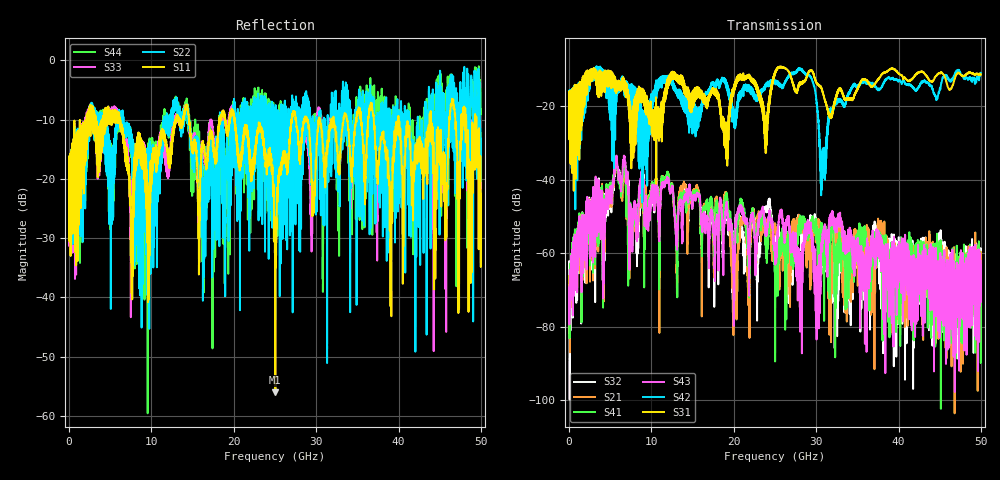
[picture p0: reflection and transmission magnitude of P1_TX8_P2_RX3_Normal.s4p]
!Keysight Technologies,N5225B,MY57041031,A.13.20.10
!Date: Friday, May 31, 2019 11:32:16
!Correction: S11(Full 4 Port(1,2,3,4))
!S12(Full 4 Port(1,2,3,4))
!S13(Full 4 Port(1,2,3,4))
!S14(Full 4 Port(1,2,3,4))
!S21(Full 4 Port(1,2,3,4))
!S22(Full 4 Port(1,2,3,4))
!S23(Full 4 Port(1,2,3,4))
!S24(Full 4 Port(1,2,3,4))
!S31(Full 4 Port(1,2,3,4))
!S32(Full 4 Port(1,2,3,4))
!S33(Full 4 Port(1,2,3,4))
!S34(Full 4 Port(1,2,3,4))
!S41(Full 4 Port(1,2,3,4))
!S42(Full 4 Port(1,2,3,4))
!S43(Full 4 Port(1,2,3,4))
!S44(Full 4 Port(1,2,3,4))
!S4P File: Measurements: <S11,S12,S13,S14>,
!<S21,S22,S23,S24>,
!<S31,S32,S33,S34>,
!<S41,S42,S43,S44>:
# Hz S  dB  R 50.0
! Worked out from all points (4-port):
!   5000 points, 10 MHz to 50 GHz, reference 50 ohm
!   strongest paths, dB at 10 MHz, 12.51 GHz, 25.01 GHz, 37.51 GHz, 50 GHz:
!     S31: -19.6, -10.8, -11.0, -12.6, -11.3
!     S42: -19.3, -14.2, -13.1, -15.6, -10.9
!     S43: -76.3, -42.0, -61.9, -55.2, -67.4
!     S41: -70.7, -41.7, -68.8, -59.2, -73.5
!     S21: -66.2, -42.0, -51.9, -52.8, -64.3
!     S32: -68.9, -41.5, -57.0, -62.4, -66.8
!   lowest |S11| = -56.0 dB at 25.05 GHz (marker M1), VSWR 1.00, Z = 49.8 - j0.000148 ohm
!   |S11| at or under -10 dB: 6.192 GHz to 12.89 GHz (6.696 GHz wide, 70.2 % of centre); 20.1 GHz to 26.99 GHz (6.893 GHz wide, 29.3 % of centre); 40 GHz to 43.77 GHz (3.764 GHz wide, 8.99 % of centre)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
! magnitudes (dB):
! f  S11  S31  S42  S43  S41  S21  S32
! 10 MHz  -19.5  -19.6  -19.3  -76.3  -70.7  -66.2  -68.9
! 5.71 GHz  -9.5  -15.2  -16.9  -34.8  -35.0  -35.4  -35.6
! 19.02 GHz  -10.7  -29.9  -13.4  -48.2  -44.2  -43.3  -47.1
! 20.11 GHz  -10.7  -13.8  -22.0  -62.3  -55.9  -68.2  -54.2
! 25.05 GHz  -56.0  -10.5  -13.0  -59.4  -71.6  -53.2  -55.4
! 30.78 GHz  -14.1  -16.1  -33.5  -56.6  -56.5  -56.4  -59.2
! 50 GHz  -22.5  -11.3  -10.9  -67.4  -73.5  -64.3  -66.8
